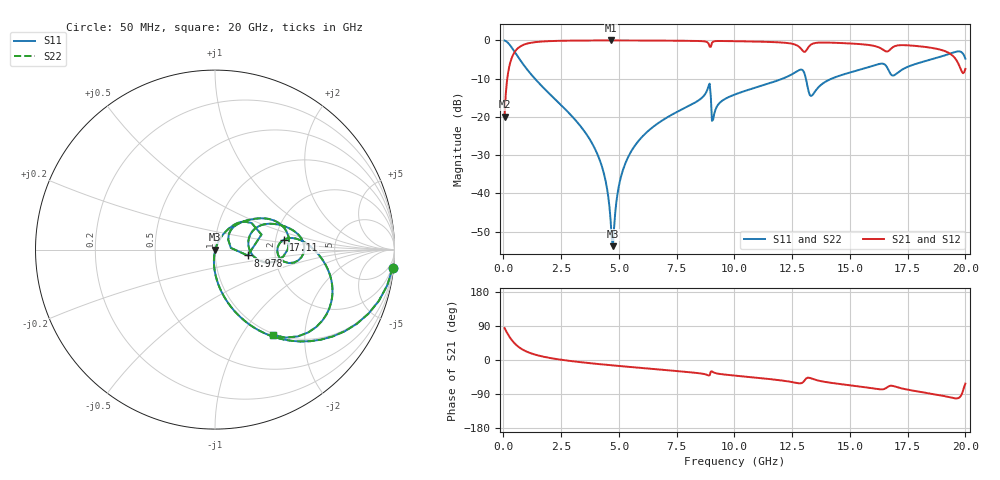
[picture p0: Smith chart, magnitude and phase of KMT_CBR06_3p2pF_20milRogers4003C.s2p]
! Data measured by Modelithics Inc. support@modelithics.com 813-866-6335
! KEMET CBR0603 3.2pF, Pad Width= 0.851mm, Pad Length= 0.64mm, Pad Gap= 0.62mm, 20mil Rogers 4003C substrate Data, January 2022
# hz S ma R 50
! 2 Port Network Data from SP1.SP block
! freq  magS11  angS11  magS21  angS21  magS12  angS12  magS22  angS22
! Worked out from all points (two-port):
!   401 points, 50 MHz to 20 GHz, reference 50 ohm
!   highest |S21| = -0.02 dB at 4.638 GHz (marker M1); lowest = -19.9 dB at 50 MHz (marker M2)
!   |S21| within 3 dB of the highest: 488.6 MHz to 19.2 GHz (18.71 GHz wide, 190 % of centre)
!   lowest |S11| = -53.8 dB at 4.738 GHz (marker M3), VSWR 1.00, Z = 50.2 + j0.0077 ohm
!   |S11| at or under -10 dB: 1.361 GHz to 12.08 GHz (10.72 GHz wide, 160 % of centre); 13.09 GHz to 14.21 GHz (1.117 GHz wide, 8.18 % of centre)
!   |S22| runs from -53.8 to 0.0 dB; largest |S21 - S12| = 0
!   S11 on the Smith chart (normalised r, x): 50 MHz: 1, -19; 8.978 GHz: 1.44, -0.10; 17.11 GHz: 2.21, +0.28; 20 GHz: 0.97, -1.39
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5e7  0.9949 -5.9  0.1009 84.0  0.1009 84.0  0.9949 -5.9
2.99375e8  0.8535 -32.3  0.5203 57.7  0.5203 57.7  0.8535 -32.3
6.485e8  0.5978 -55.2  0.8007 34.8  0.8007 34.8  0.5978 -55.2
1.496375e9  0.2853 -77.7  0.9572 12.1  0.9572 12.1  0.2853 -77.7
3.391625e9  0.07216 -94.8  0.9956 -6.1  0.9956 -6.1  0.07216 -94.8
4.2395e9  0.02372 -96.9  0.9977 -11.4  0.9977 -11.4  0.02372 -96.9
4.6385e9  0.004528 -78.3  0.9979 -13.7  0.9979 -13.7  0.004528 -78.3
4.73825e9  0.002051 2.1  0.9979 -14.3  0.9979 -14.3  0.002051 2.1
5.0375e9  0.0143 65.9  0.9977 -16.0  0.9977 -16.0  0.0143 65.9
5.33675e9  0.02728 68.0  0.9973 -17.6  0.9973 -17.6  0.02728 68.0
6.73325e9  0.08434 63.3  0.9938 -25.0  0.9938 -25.0  0.08434 63.3
8.828e9  0.227 43.4  0.9457 -39.4  0.9457 -39.4  0.227 43.4
8.977625e9  0.1851 -10.2  0.824 -30.5  0.824 -30.5  0.1851 -10.2
9.12725e9  0.1102 46.3  0.9743 -33.5  0.9743 -33.5  0.1102 46.3
1.0025e10  0.1968 47.6  0.976 -41.3  0.976 -41.3  0.1968 47.6
1.286788e10  0.4159 10.3  0.7881 -61.5  0.7881 -61.5  0.4159 10.3
1.336662e10  0.1914 14.0  0.8992 -49.5  0.8992 -49.5  0.1914 14.0
1.526188e10  0.4007 19.3  0.9023 -68.7  0.9023 -68.7  0.4007 19.3
1.670825e10  0.3884 -9.8  0.7417 -68.7  0.7417 -68.7  0.3884 -9.8
1.710725e10  0.3861 8.1  0.8628 -72.8  0.8628 -72.8  0.3861 8.1
1.945138e10  0.6898 -18.4  0.6303 -100.2  0.6303 -100.2  0.6898 -18.4
2e10  0.5757 -55.9  0.4251 -62.3  0.4251 -62.3  0.5757 -55.9
